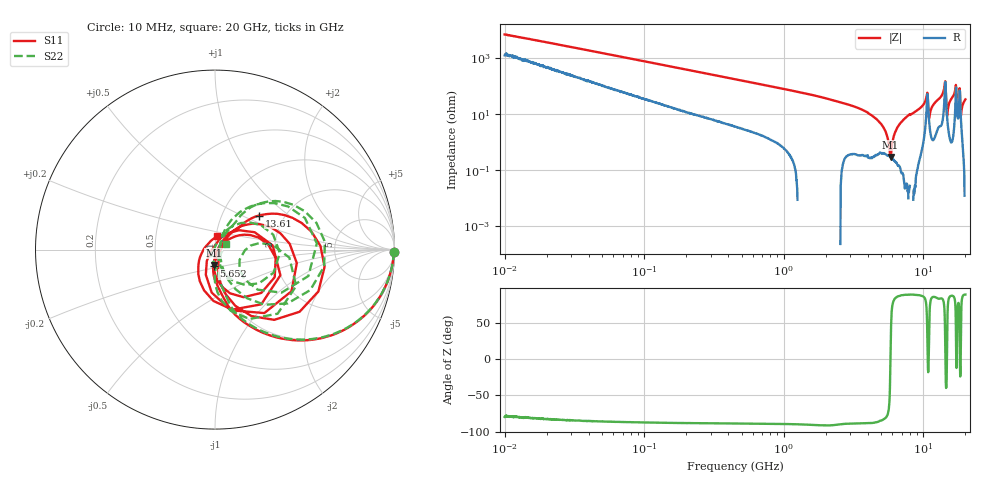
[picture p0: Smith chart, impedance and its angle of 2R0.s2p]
!Keysight Technologies,P5008B,MY61100088,A.16.20.02
!Date: Monday, October 30, 2023 15:09:54
!Correction: S11(C  2-Port  )
!S21(C  2-Port  )
!S12(C  2-Port  )
!S22(C  2-Port  )
!S2P File: Measurements: S11, S21, S12, S22:Log Frequency Sweep
# Hz S  dB  R 50
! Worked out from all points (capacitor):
!   1601 points, 10 MHz to 20 GHz, reference 50 ohm
!   read as one part in series: C = 2.19 pF near 10.39 MHz
!   lowest |Z| = 298 mohm at 5.816 GHz (marker M1)
!   series resonance near 5.812 GHz, so ESL is about 340 pH
!   S11 on the Smith chart (normalised r, x): 10 MHz: open; 5.652 GHz: 0.97, -0.18; 13.61 GHz: 1.49, +0.63; 20 GHz: 1.01, +0.15
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1e7  -0.02 -0.8  -37.18 79.0  -37.19 78.9  -0.02 -0.8
3.555162e7  -0.04 -2.7  -26.77 82.5  -26.76 82.5  -0.04 -2.7
1.263918e8  -0.16 -9.2  -16.14 78.6  -16.14 78.6  -0.16 -9.1
4.472136e8  -1.23 -29.4  -6.39 59.6  -6.40 59.6  -1.23 -29.1
1.589917e9  -6.73 -66.1  -0.98 25.2  -0.99 25.2  -6.73 -65.0
5.652411e9  -20.75 -95.1  -0.04 -4.3  -0.05 -4.3  -20.75 -86.9
5.815842e9  -21.35 -94.5  -0.04 -5.0  -0.04 -4.9  -21.33 -88.5
8.344716e9  -28.94 -88.5  0.01 -14.3  0.01 -14.3  -29.86 -116.4
9.30816e9  -35.74 -36.1  0.01 -18.4  0.01 -18.4  -44.37 -175.8
9.622897e9  -32.51 14.8  -0.00 -20.1  -0.01 -20.1  -35.75 86.9
1.053187e10  -11.98 15.4  -1.33 -32.6  -1.33 -32.6  -12.22 38.2
1.083639e10  -11.78 -71.0  -1.66 -9.0  -1.67 -9.0  -11.75 -49.5
1.130974e10  -28.54 -88.9  -0.13 -18.7  -0.13 -18.7  -27.24 -63.8
1.163675e10  -31.21 36.2  -0.07 -21.9  -0.08 -21.9  -30.28 34.3
1.361179e10  -10.19 37.8  -0.80 -37.3  -0.80 -37.3  -10.14 49.6
1.427404e10  -4.18 -8.9  -6.60 -44.3  -6.60 -44.3  -4.24 4.0
1.482695e10  -16.75 -82.1  -0.60 -14.7  -0.61 -14.7  -17.38 -67.9
1.540129e10  -22.13 43.0  -0.16 -27.3  -0.17 -27.3  -21.17 61.1
1.661757e10  -10.89 29.7  -0.79 -43.9  -0.80 -43.9  -10.15 50.6
1.767617e10  -32.89 90.5  -0.79 -31.9  -0.80 -31.9  -16.17 -10.3
1.862442e10  -14.18 -115.7  -0.78 -21.9  -0.79 -21.9  -12.47 -86.7
2e10  -22.53 81.6  -0.05 -38.4  -0.06 -38.4  -23.47 25.5
